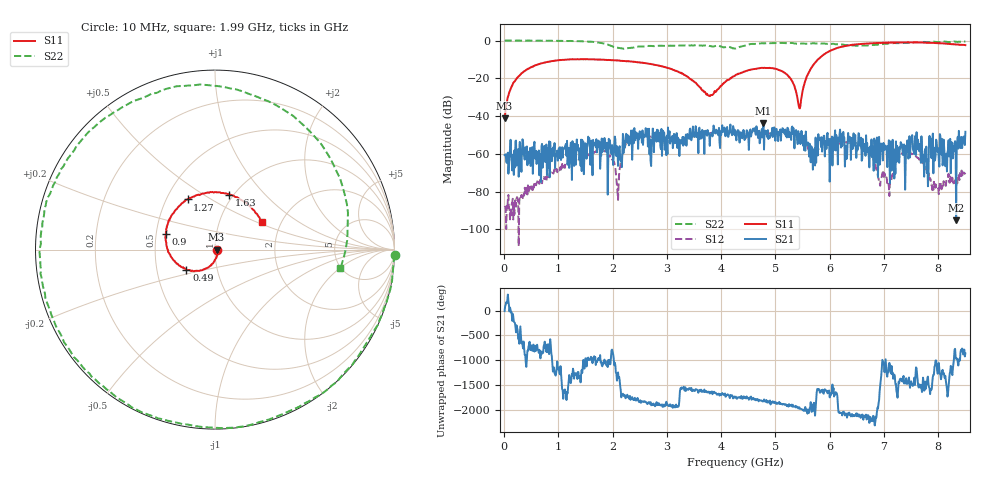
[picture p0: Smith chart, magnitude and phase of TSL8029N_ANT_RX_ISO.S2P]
!Agilent Technologies,E5071C,MY46523237,B.13.01
!Date: Wed Aug 16 14:10:31 2023
!Data & Calibration Information:
!Freq	S11:SOLT2(ON)	S21:SOLT2(ON)	S12:SOLT2(ON)	S22:SOLT2(ON)
!PortZ  Port1:50+j0  Port2:50+j0
!Above PortZ is port z conversion or system Z0 setting when saving the data.
!When reading, reference impedance value at option line is always used.
# Hz S dB R 50
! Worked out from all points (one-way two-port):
!   850 points, 10 MHz to 8.5 GHz, reference 50 ohm
!   highest |S21| = -43.68 dB at 4.78 GHz (marker M1); lowest = -95.2 dB at 8.33 GHz (marker M2)
!   lowest |S11| = -41.2 dB at 10 MHz (marker M3), VSWR 1.02, Z = 50.9 - j0.108 ohm
!   |S11| at or under -10 dB: start of sweep to 1.204 GHz; 1.673 GHz to 1.697 GHz (23.82 MHz wide, 1.41 % of centre); 1.705 GHz to 5.785 GHz (4.08 GHz wide, 109 % of centre)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
!   |S22| runs from -4.3 to 0.0 dB; largest |S21 - S12| = 0.0043
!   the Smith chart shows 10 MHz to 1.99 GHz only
!   S11 on the Smith chart (normalised r, x): 10 MHz: 1.02, -0.00; 490 MHz: 0.71, -0.16; 900 MHz: 0.56, +0.10; 1.27 GHz: 0.64, +0.40; 1.63 GHz: 0.96, +0.65; 1.99 GHz: 1.59, +0.54
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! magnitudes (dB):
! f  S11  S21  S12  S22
! 10 MHz  -41.2  -60.6  -87.6  0.0
! 490 MHz  -14.2  -66.4  -79.1  -0.1
! 900 MHz  -10.9  -59.6  -70.0  -0.2
! 1.27 GHz  -9.9  -55.4  -64.0  -0.3
! 1.43 GHz  -9.9  -69.1  -62.8  -0.4
! 1.63 GHz  -10.0  -71.3  -59.2  -0.7
! 1.99 GHz  -10.4  -55.3  -63.0  -3.0
! 2.1 GHz  -10.6  -66.4  -84.4  -3.8
! 2.33 GHz  -11.1  -54.5  -51.2  -3.9
! 2.84 GHz  -13.2  -47.5  -52.4  -2.8
! 3.79 GHz  -29.4  -55.7  -49.1  -2.9
! 4.26 GHz  -18.4  -50.3  -49.0  -4.3
! 4.78 GHz  -14.6  -43.7  -48.5  -1.5
! 5.22 GHz  -18.1  -46.2  -48.9  -1.3
! 5.44 GHz  -35.7  -49.4  -50.0  -1.7
! 5.67 GHz  -14.1  -56.6  -61.0  -1.5
! 6.49 GHz  -2.0  -62.1  -54.1  -2.7
! 7.09 GHz  -1.1  -52.8  -77.3  -1.5
! 7.42 GHz  -1.0  -59.1  -58.6  -1.2
! 7.97 GHz  -1.4  -53.3  -78.7  -0.8
! 8.33 GHz  -2.1  -95.2  -76.2  -0.7
! 8.5 GHz  -2.4  -48.3  -70.8  -0.6
